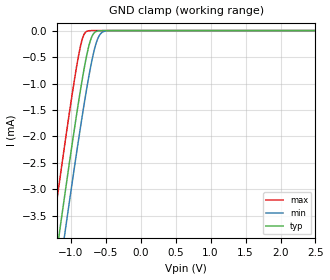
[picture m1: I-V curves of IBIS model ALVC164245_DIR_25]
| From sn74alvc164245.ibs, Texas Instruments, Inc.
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[Model]   ALVC164245_DIR_25
Model_type  Input
Vinl=0.7
Vinh=1.7
| variable   typ   min   max
C_comp   6.5pF   NA   NA
[Temperature Range]   40   100   -40
| Ambient temperature   25   85   -40
[Voltage range]   2.5   2.3   2.7
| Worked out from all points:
|   GND clamp passes 1 mA (typ) near -0.85 V on its own axis
[GND Clamp]
| ALVC164245_DIR_25
|   Voltage   I(typ)   I(min)   I(max)
-2.5V     -16.88mA   -17.58mA   -15.98mA
-1.285V   -4.967mA   -5.705mA   -4.014mA
-1.25V    -4.634mA   -5.373mA   -3.679mA
-1.155V   -3.736mA   -4.476mA   -2.78mA
-1.075V   -2.991mA   -3.73mA    -2.037mA
-880mV    -1.265mA   -1.975mA   -406.2uA
-830mV    -866.7uA   -1.551mA   -133.3uA
-780mV    -510.2uA   -1.147mA   -20.22uA
-710mV    -148.5uA   -636.7uA   -739.2nA
-640mV    -18.77uA   -246.3uA   -24.69nA
-515mV    -217.6nA   -11.23uA   -63.37pA
2.5V      4.712pA    817.5pA    4.189pA
